| IBIS file stm32mp157xab_lfbga354.ibs
[IBIS ver]   4.2
[File name]   stm32mp157xab_lfbga354.ibs
[File Rev]   2.2
[Date]   07-07-2026
[Source]   Data Created at STMicroelectronics
[Disclaimer]  This information is for modeling purpose only and is
   not guaranted.
   The information is subject to change without notice.
[Copyright]   Copyright 2026 STMicroelectronics Inc.
|   Component stm32mp157xab_lfbga354
[Component] stm32mp157xab_lfbga354
[Manufacturer] STMicroelectronics
[Package]
| variable   typ   min   max
R_pkg  5.94E-01  2.68E-01  8.52E-01
L_pkg  3.75E-09  1.99E-09  5.34E-09
C_pkg  1.24E-12  9.33E-13  5.22E-12
[Pin]   signal_name   model_name
A1  VSS  gnd
A2  PG15  io8_ft_hslv
A3  PD0  io8_ft_hslv
A4  PD1  io8_ft_hslv
A5  PE3  io8_ft_hslv
A6  PG6  io8_ft_hslv
A7  PB3  io8_ft_hslv
A8  PB15  io8_ft_hslv
A9  PC7  io8_ft_hslv
A10  PC9  io8_ft_hslv
A11  PC11  io8_ft_hslv
A12  VDD_Unused  nc
A13  DNU  nc
A14  DNU  nc
A15  DNU  nc
A16  VDD1V2_Unused  nc
A17  DDR_DQ0  PDDRIO_PAD
A18  DDR_DQ1  PDDRIO_PAD
A19  VSS  gnd
B1  PE1  io8_ft
B2  VSS  gnd
B3  PE6  io8_ft_hslv
B4  PD7  io8_ft_hslv
B5  PB7  io8_ft_hslv
B6  VSS  gnd
B7  PE5  io8_ft_hslv
B8  PA8  io8_ft_hslv
B9  PB4  io8_ft_hslv
B10  PD2  io8_ft_hslv
B11  PE4  io8_ft_hslv
B12  VDDA1V8_Unused  nc
B13  DNU  nc
B14  DNU  nc
B15  DNU  nc
B16  VDD1V2_Unused  nc
B17  DDR_DQ3  PDDRIO_PAD
B18  DDR_DQ7  PDDRIO_PAD
B19  DDR_DQS0N  PDIFF_PAD
C1  PE11  io8_ft
C2  PE13  io8_ft_hslv
C3  VSS  gnd
C4  PE0  io8_ft_hslv
C5  PD10  io8_ft_hslv
C6  PD3  io8_ft_hslv
C7  PA15  io8_ft_hslv
C8  PA9  io8_ft_hslv
C9  PB14  io8_ft_hslv
C10  PC12  io8_ft_hslv
C11  PC8  io8_ft_hslv
C12  VSS  nc
C13  VSS  nc
C14  VSS  nc
C15  VSS  nc
C16  VSS  nc
C17  VSS  gnd
C18  DDR_DQM0  PDDRIO_PAD
C19  DDR_DQS0P  PDIFF_PAD
D1  VSS  gnd
D2  PE12  io8_ft_hslv
D3  PE14  io8_ft_hslv
D4  VSS  gnd
D5  VSS  gnd
D6  PD4  io8_ft_hslv
D7  PD5  io8_ft_hslv
D8  VSS  gnd
D9  PB9  io8_ft_hslv
D10  PC6  io8_ft_hslv
D11  PC10  io8_ft_hslv
D12  NJTRST  isudqf
D13  JTDI  isudqf
D14  JTDO-TRACESWO  io8_ft
D15  JTMS-SWDIO  io8_ft
D16  JTCK-SWCLK  isudqf
D17  DDR_DQ5  PDDRIO_PAD
D18  DDR_DQ2  PDDRIO_PAD
D19  DDR_DQ6  PDDRIO_PAD
E1  PE15  io8_ft
E2  VSS  gnd
E3  PD6  io8_ft_hslv
E4  VSS  gnd
E5  VSS  gnd
E6  VSS  gnd
E7  VDDCORE  power
E8  VSS  gnd
E9  VDDCORE  power
E10  VSS  gnd
E11  VDDCORE  power
E12  VSS  gnd
E13  VDDCORE  power
E14  VSS  gnd
E15  VDDQ_DDR  power
E16  VSS  gnd
E17  DDR_A7  PDDRIO_PAD
E18  DDR_DQ4  PDDRIO_PAD
F1  PG12  io8_ft_hslv
F2  PD8  io8_ft
F3  PD14  io8_ft
F4  VDDCORE  power
F5  VSS  gnd
F6  VDDCORE  power
F7  VSS  gnd
F8  VDDCORE  power
F9  VSS  gnd
F10  VDDCORE  power
F11  VSS  gnd
F12  VDDCORE  power
F13  VSS_PLL2  gnd
F14  VDDQ_DDR  power
F15  VSS  gnd
F17  DDR_A13  PDDRIO_PAD
F18  DDR_ZQ  nc
F19  DDR_A3  PDDRIO_PAD
G1  PD15  io8_ft
G2  VSS  gnd
G3  PD9  io8_ft
G4  VSS  gnd
G5  VDDCORE  power
G6  VSS  gnd
G7  VDDCORE  power
G8  VSS  gnd
G9  VDDCORE  power
G10  VSS  gnd
G11  VDDCORE  power
G12  VSS  gnd
G13  VDD_PLL2  power
G14  VSS  gnd
G15  VDDQ_DDR  power
G16  DDR_RESETN  PDDRIO_PAD
G17  DDR_A9  PDDRIO_PAD
G18  DDR_A2  PDDRIO_PAD
G19  DDR_BA0  PDDRIO_PAD
H1  PC14-OSC32_IN  io8_ft
H2  PC15-OSC32_OUT  io8_ft
H3  VBAT  power
H4  VDDCORE  power
H5  VSS  gnd
H6  VDDCORE  power
H7  VSS  gnd
H8  VDDCORE  power
H9  VSS  gnd
H10  VDDCORE  power
H11  VSS  gnd
H12  VDDCORE  power
H13  VSS  gnd
H14  VDDQ_DDR  power
H15  VSS  gnd
H17  DDR_A5  PDDRIO_PAD
H18  DDR_A0  PDDRIO_PAD
H19  DDR_ODT  PDDRIO_PAD
|J1  NRST  ioreset_ft_v33
J1  NRST  nc
J2  NRST_CORE  isudqf
J3  VSS  gnd
J4  VSS_PLL  gnd
J5  VDD_PLL  power
J6  VSS  gnd
J7  VDDCORE  power
J8  VSS  gnd
J9  VDDCORE  power
J10  VSS  gnd
J11  VDDCORE  power
J12  VSS  gnd
J13  VDDCORE  power
J14  VSS  gnd
J15  VDDQ_DDR  power
J16  DDR_BA2  PDDRIO_PAD
J17  DDR_WEN  PDDRIO_PAD
J18  DDR_CSN  PDDRIO_PAD
J19  DDR_DTO1  PDDRIO_PAD
K1  BOOT0  isudqf
K2  VSS  gnd
K3  PC13  io8_ft
K4  BOOT1  isudqf
K5  VSS  gnd
K6  VDD  power
K7  VSS  gnd
K8  VDDCORE  power
K9  VSS  gnd
K10  VDDCORE  power
K11  VSS  gnd
K12  VDDCORE  power
K13  VSS  gnd
K14  VDDQ_DDR  power
K15  VSS  gnd
K17  DDR_CASN  PDDRIO_PAD
K18  DDR_DTO0  PDDRIO_PAD
K19  DDR_CLKN  PDDRIO_PAD
L1  PWR_ON  io8_ft
L2  BOOT2  isudqf
L3  VDD_ANA  nc
L4  VSS_ANA  nc
L5  VDD  power
L6  VSS  gnd
L7  VDD  power
L8  VSS  gnd
L9  VDDCORE  power
L10  VSS  gnd
L11  VDDCORE  power
L12  VSS  gnd
L13  VDDCORE  power
L14  VSS  gnd
L15  VDDQ_DDR  power
L16  DDR_A15  PDDRIO_PAD
L17  DDR_A12  PDDRIO_PAD
L18  DDR_RASN  PDDRIO_PAD
L19  DDR_CLKP  PDDRIO_PAD
M1  PH0-OSC_IN  io8_ft
M2  PH1-OSC_OUT  io8_ft
M3  VREF-  nc
M4  VDDA  nc
M5  VSS  gnd
M6  VDD  power
M7  VSS  gnd
M8  VDD  power
M9  VSS  gnd
M10  VDDCORE  power
M11  VSS  gnd
M12  VDDCORE  power
M13  VSS  gnd
M14  VDDQ_DDR  power
M15  VSS  gnd
M17  DDR_A1  PDDRIO_PAD
M18  DDR_A11  PDDRIO_PAD
M19  DDR_A10  PDDRIO_PAD
N1  PDR_ON_CORE  isudqf
N2  PDR_ON  isudqf
N3  VREF+  nc
N4  VSSA  gnd
N5  VDD  power
N6  VSS  gnd
N7  VDD  power
N8  VSS  gnd
N9  VDD  power
N10  VSS  gnd
N11  VDDCORE  power
N12  VSS  gnd
N13  VDDCORE  power
N14  VSS  gnd
N15  VDDQ_DDR  power
N16  DDR_A6  PDDRIO_PAD
N17  DDR_BA1  PDDRIO_PAD
N18  DDR_A14  PDDRIO_PAD
N19  DDR_ATO  nc
P1  PWR_LP  io8_ft
P2  PA13  io8_ft
P3  PA3  io8_ft
P4  PA5  io8_ft_hslv
P5  VSSA  gnd
P6  VDD  power
P7  VSS  gnd
P8  VDD  power
P9  VSS  gnd
P10  VDD  power
P11  VSS  gnd
P12  VDDCORE  power
P13  VSS  gnd
P14  VDDQ_DDR  power
P15  VSS  gnd
P17  DDR_A4  PDDRIO_PAD
P18  DDR_DQ8  PDDRIO_PAD
P19  DDR_CKE  PDDRIO_PAD
R1  PA14  io8_ft
R2  VSS  gnd
R3  PA0  io8_ft_hslv
R4  PA4  io8_ft
R5  VSSA  gnd
R6  VSS  gnd
R7  VDD_OTP  power
R8  VSS  gnd
R9  VDD  power
R10  VSS  gnd
R11  VDD  power
R12  VSS  gnd
R13  VDDCORE  power
R14  VSS  gnd
R15  VDDQ_DDR  power
R16  VSS  gnd
R17  DDR_A8  PDDRIO_PAD
R18  DDR_DQ10  PDDRIO_PAD
T1  PE2  io8_ft_et_i2c_hslv
T2  PC2  io8_ft_hslv_et
T3  PC3  io8_ft_hslv
T4  VSS  gnd
T5  PA6  io8_ft_hslv
T6  PA7  io8_ft_hslv
T7  PC0  io8_ft_hslv
T8  PB5  io8_ft_hslv_et
T9  PB13  io8_ft_hslv_et
T10  PE7  io8_ft_hslv
T11  PE8  io8_ft_hslv
T12  PB6  io8_ft_i2c_hslv
T13  PB2  io8_ft_hslv
T14  PG9  io8_ft_hslv
T15  BYPASS_REG1V8  isudqf
T16  PA10  io8usb_id_otg20_ft
T17  DDR_DQ9  PDDRIO_PAD
T18  DDR_DQ13  PDDRIO_PAD
T19  DDR_DQS1N  PDIFF_PAD
U1  PG14  io8_ft_hslv_et
U2  PG13  io8_ft_hslv_et
U3  VSS  gnd
U4  PA1  io8_ft_hslv
U5  PF11  io8_ft_hslv
U6  VSS  gnd
U7  PG8  io8_ft_hslv_et
U8  VSS  gnd
U9  PF10  io8_ft_hslv
U10  PF8  io8_ft_hslv
U11  PD12  io8_ft_i2c_hslv
U12  PD13  io8_ft_i2c_hslv
U13  VSS_USBHS  nc
U14  VSS_USBHS  nc
U15  OTG_VBUS  io8usb_vbus_otg20_ft
U16  PA12  io8_i2c_usb_lsfs_bcd_otg20_ft
U17  VSS  gnd
U18  DDR_DM1  PDDRIO_PAD
U19  DDR_DQS1P  PDIFF_PAD
V1  PB11  io8_ft_et_i2c_hslv
V2  PC1  io8_ft_hslv
V3  PB1  io8_ft
V4  PC5  io8_ft
V5  PB12  io8_ft_hslv_et
V6  PG11  io8_ft_hslv_et
V7  PG10  io8_ft_hslv
V8  PD11  io8_ft_hslv
V9  PF6  io8_ft_hslv
V10  PE10  io8_ft_hslv
V11  VDDA1V8_REG  nc
V12  VSS_USBHS  nc
V13  USB_DM2  nc
V14  USB_DP1  nc
V15  VSS_USBHS  nc
V16  USB_RREF  nc
V17  PA11  io8_i2c_usb_lsfs_bcd_otg20_ft
V18  DDR_DQ14  PDDRIO_PAD
V19  DDR_DQ11  PDDRIO_PAD
W1  VSS  gnd
W2  PA2  io8_ft_hslv
W3  PB0  io8_ft
W4  PC4  io8_ft
W5  PB10  io8_ft_i2c_hslv
W6  PB8  io8_ft_et_i2c_hslv
W7  PE9  io8_ft_hslv
W8  PF7  io8_ft_hslv
W9  PF9  io8_ft_hslv
W10  PG7  io8_ft_hslv
W11  VDDA1V1_REG  nc
W12  VDD3V3_USBHS  power
W13  USB_DP2  nc
W14  USB_DM1  nc
W15  VDD3V3_USBFS  power
W16  DDR_VREF  POWER
W17  DDR_DQ15  PDDRIO_PAD
W18  DDR_DQ12  PDDRIO_PAD
W19  VSS  gnd
[Package Model]   500-lfbga-16x16-354-100mhz-181019
[Pin Mapping]   pulldown_ref   pullup_ref   | Comment
A1  VSS  nc
A2  VSS  VDD
A3  VSS  VDD
A4  VSS  VDD
A5  VSS  VDD
A6  VSS  VDD
A7  VSS  VDD
A8  VSS  VDD
A9  VSS  VDD
A10  VSS  VDD
A11  VSS  VDD
A12  nc  nc
A13  nc nc
A14  nc nc
A15  nc nc
A16  nc nc
A17  VSS  VDDQ_DDR
A18  VSS  VDDQ_DDR
A19  VSS  nc
B1  VSS  VDD
B2  VSS  nc
B3  VSS  VDD
B4  VSS  VDD
B5  VSS  VDD
B6  VSS  nc
B7  VSS  VDD
B8  VSS  VDD
B9  VSS  VDD
B10  VSS  VDD
B11  VSS  VDD
B12  nc nc
B13  nc nc
B14  nc nc
B15  nc nc
B16  nc  nc
B17  VSS  VDDQ_DDR
B18  VSS  VDDQ_DDR
B19  VSS  VDDQ_DDR
C1  VSS  VDD
C2  VSS  VDD
C3  VSS  nc
C4  VSS  VDD
C5  VSS  VDD
C6  VSS  VDD
C7  VSS  VDD
C8  VSS  VDD
C9  VSS  VDD
C10  VSS  VDD
C11  VSS  VDD
C12  nc nc
C13  nc nc
C14  nc nc
C15  nc nc
C16  nc nc
C17  VSS  nc
C18  VSS  VDDQ_DDR
C19  VSS  VDDQ_DDR
D1  VSS  nc
D2  VSS  VDD
D3  VSS  VDD
D4  VSS  nc
D5  VSS  nc
D6  VSS  VDD
D7  VSS  VDD
D8  VSS  nc
D9  VSS  VDD
D10  VSS  VDD
D11  VSS  VDD
D12  VSS  VDD
D13  VSS  VDD
D14  VSS  VDD
D15  VSS  VDD
D16  VSS  VDD
D17  VSS  VDDQ_DDR
D18  VSS  VDDQ_DDR
D19  VSS  VDDQ_DDR
E1  VSS  VDD
E2  VSS  nc
E3  VSS  VDD
E4  VSS  nc
E5  VSS  nc
E6  VSS  nc
E7  nc  vddcore
E8  VSS  nc
E9  nc  vddcore
E10  VSS  nc
E11  nc  vddcore
E12  VSS  nc
E13  nc  vddcore
E14  VSS  nc
E15  nc  VDDQ_DDR
E16  VSS  nc
E17  VSS  VDDQ_DDR
E18  VSS  VDDQ_DDR
F1  VSS  VDD
F2  VSS  VDD
F3  VSS  VDD
F4  nc  vddcore
F5  VSS  nc
F6  nc  vddcore
F7  VSS  nc
F8  nc  vddcore
F9  VSS  nc
F10  nc  vddcore
F11  VSS  nc
F12  nc  vddcore
F13  VSS  nc
F14  nc  VDDQ_DDR
F15  VSS  nc
F17  VSS  VDDQ_DDR
F18  nc nc
F19  VSS  VDDQ_DDR
G1  VSS  VDD
G2  VSS  nc
G3  VSS  VDD
G4  VSS  nc
G5  nc  vddcore
G6  VSS  nc
G7  nc  vddcore
G8  VSS  nc
G9  nc  vddcore
G10  VSS  nc
G11  nc  vddcore
G12  VSS  nc
G13  nc  VDD
G14  VSS  nc
G15  nc  VDDQ_DDR
G16  VSS  VDDQ_DDR
G17  VSS  VDDQ_DDR
G18  VSS  VDDQ_DDR
G19  VSS  VDDQ_DDR
H1  nc  nc
H2  nc  nc
H3  nc  VDD_sw
H4  nc  vddcore
H5  VSS  nc
H6  nc  vddcore
H7  VSS  nc
H8  nc  vddcore
H9  VSS  nc
H10  nc  vddcore
H11  VSS  nc
H12  nc  vddcore
H13  VSS  nc
H14  nc  VDDQ_DDR
H15  VSS  nc
H17  VSS  VDDQ_DDR
H18  VSS  VDDQ_DDR
H19  VSS  VDDQ_DDR
J1  nc  nc
J2  VSS  VDD
J3  VSS  nc
J4  VSS  nc
J5  nc  VDD
J6  VSS  nc
J7  nc  vddcore
J8  VSS  nc
J9  nc  vddcore
J10  VSS  nc
J11  nc  vddcore
J12  VSS  nc
J13  nc  vddcore
J14  VSS  nc
J15  nc  VDDQ_DDR
J16  VSS  VDDQ_DDR
J17  VSS  VDDQ_DDR
J18  VSS  VDDQ_DDR
J19  VSS  VDDQ_DDR
K1  VSS  VDD
K2  VSS  nc
K3  nc  nc
K4  VSS  VDD
K5  VSS  nc
K6  nc  VDD
K7  VSS  nc
K8  nc  vddcore
K9  VSS  nc
K10  nc  vddcore
K11  VSS  nc
K12  nc  vddcore
K13  VSS  nc
K14  nc  VDDQ_DDR
K15  VSS  nc
K17  VSS  VDDQ_DDR
K18  VSS  VDDQ_DDR
K19  VSS  VDDQ_DDR
L1  VSS  VDD
L2  VSS  VDD
L3  nc nc
L4  nc nc
L5  nc  VDD
L6  VSS  nc
L7  nc  VDD
L8  VSS  nc
L9  nc  vddcore
L10  VSS  nc
L11  nc  vddcore
L12  VSS  nc
L13  nc  vddcore
L14  VSS  nc
L15  nc  VDDQ_DDR
L16  VSS  VDDQ_DDR
L17  VSS  VDDQ_DDR
L18  VSS  VDDQ_DDR
L19  VSS  VDDQ_DDR
M1  VSS  VDD
M2  VSS  VDD
M3  nc nc
M4  nc nc
M5  VSS  nc
M6  nc  VDD
M7  VSS  nc
M8  nc  VDD
M9  VSS  nc
M10  nc  vddcore
M11  VSS  nc
M12  nc  vddcore
M13  VSS  nc
M14  nc  VDDQ_DDR
M15  VSS  nc
M17  VSS  VDDQ_DDR
M18  VSS  VDDQ_DDR
M19  VSS  VDDQ_DDR
N1  VSS  VDD
N2  VSS  VDD
N3  nc nc
N4  VSS  nc
N5  nc  VDD
N6  VSS  nc
N7  nc  VDD
N8  VSS  nc
N9  nc  VDD
N10  VSS  nc
N11  nc  vddcore
N12  VSS  nc
N13  nc  vddcore
N14  VSS  nc
N15  nc  VDDQ_DDR
N16  VSS  VDDQ_DDR
N17  VSS  VDDQ_DDR
N18  VSS  VDDQ_DDR
N19  nc nc
P1  VSS  VDD
P2  VSS  VDD
P3  VSS  VDD
P4  VSS  VDD
P5  VSS  nc
P6  nc  VDD
P7  VSS  nc
P8  nc  VDD
P9  VSS  nc
P10  nc  VDD
P11  VSS  nc
P12  nc  vddcore
P13  VSS  nc
P14  nc  VDDQ_DDR
P15  VSS  nc
P17  VSS  VDDQ_DDR
P18  VSS  VDDQ_DDR
P19  VSS  VDDQ_DDR
R1  VSS  VDD
R2  VSS  nc
R3  VSS  VDD
R4  VSS  VDD
R5  VSS  nc
R6  VSS  nc
R7  nc  VDD
R8  VSS  nc
R9  nc  VDD
R10  VSS  nc
R11  nc  VDD
R12  VSS  nc
R13  nc  vddcore
R14  VSS  nc
R15  nc  VDDQ_DDR
R16  VSS  nc
R17  VSS  VDDQ_DDR
R18  VSS  VDDQ_DDR
T1  VSS  VDD
T2  VSS  VDD
T3  VSS  VDD
T4  VSS  nc
T5  VSS  VDD
T6  VSS  VDD
T7  VSS  VDD
T8  VSS  VDD
T9  VSS  VDD
T10  VSS  VDD
T11  VSS  VDD
T12  VSS  VDD
T13  VSS  VDD
T14  VSS  VDD
T15  VSS  VDD
T16  VSS  vddusbls  | Depending on IO usage
| T16  VSS  VDD  | Depending on IO usage
T17  VSS  VDDQ_DDR
T18  VSS  VDDQ_DDR
T19  VSS  VDDQ_DDR
U1  VSS  VDD
U2  VSS  VDD
U3  VSS  nc
U4  VSS  VDD
U5  VSS  VDD
U6  VSS  nc
U7  VSS  VDD
U8  VSS  nc
U9  VSS  VDD
U10  VSS  VDD
U11  VSS  VDD
U12  VSS  VDD
U13  nc nc
U14  nc nc
U15  VSS  vddusbls  | Depending on IO usage
| U15  VSS  VDD  | Depending on IO usage
U16  VSS  vddusbls  | Depending on IO usage
| U16  VSS  VDD  | Depending on IO usage
U17  VSS  nc
U18  VSS  VDDQ_DDR
U19  VSS  VDDQ_DDR
V1  VSS  VDD
V2  VSS  VDD
V3  VSS  VDD
V4  VSS  VDD
V5  VSS  VDD
V6  VSS  VDD
V7  VSS  VDD
V8  VSS  VDD
V9  VSS  VDD
V10  VSS  VDD
V11  nc  nc
V12  nc nc
V13  nc nc
V14  nc nc
V15  nc nc
V16  nc nc
V17  VSS  vddusbls  | Depending on IO usage
| V17  VSS  VDD  | Depending on IO usage
V18  VSS  VDDQ_DDR
V19  VSS  VDDQ_DDR
W1  VSS  nc
W2  VSS  VDD
W3  VSS  VDD
W4  VSS  VDD
W5  VSS  VDD
W6  VSS  VDD
W7  VSS  VDD
W8  VSS  VDD
W9  VSS  VDD
W10  VSS  VDD
W11  nc  nc
W12  nc  vddusbhs
W13  nc nc
W14  nc nc
W15  nc  vddusbls
W16  nc  VDDQ_DDR
W17  VSS  VDDQ_DDR
W18  VSS  VDDQ_DDR
W19  VSS  nc
|**********************DIFF PIN*********************************************
[Diff_pin]   inv_pin   vdiff   tdelay_typ   tdelay_min   tdelay_max
   L19   K19   0.320V   0ns   NA   NA   |CK
   C19   B19   0.320V   0ns   NA   NA   |DQS0
   U19   T19   0.320V   0ns   NA   NA   |DQS1
[Model Selector] io8usb_id_otg20_ft
io8_ft_ls_1v2   "GPIO - 5V tolerant - 1.2V range - Low speed"
io8_ft_ms_1v2   "GPIO - 5V tolerant - 1.2V range - Med speed"
io8_ft_hs_1v2   "GPIO - 5V tolerant - 1.2V range - High speed"
io8_ft_fs_1v2   "GPIO - 5V tolerant - 1.2V range - Fast speed"
io8_ft_hs_1v8   "GPIO - 5V tolerant - 1.8V range - High speed"
io8_ft_fs_1v8   "GPIO - 5V tolerant - 1.8V range - Fast speed"
io8_ft_ms_1v8   "GPIO - 5V tolerant - 1.8V range - Med speed"
io8_ft_ls_1v8   "GPIO - 5V tolerant - 1.8V range - Low speed"
io8_ft_hs_3v3   "GPIO - 5V tolerant - 3.3V range - High speed"
io8_ft_fs_3v3   "GPIO - 5V tolerant - 3.3V range - Fast speed"
io8_ft_ms_3v3   "GPIO - 5V tolerant - 3.3V range - Med speed"
io8_ft_ls_3v3   "GPIO - 5V tolerant - 3.3V range - Low speed"
[Model Selector] io8usb_vbus_otg20_ft
io8_ft_ls_1v2   "GPIO - 5V tolerant - 1.2V range - Low speed"
io8_ft_ms_1v2   "GPIO - 5V tolerant - 1.2V range - Med speed"
io8_ft_hs_1v2   "GPIO - 5V tolerant - 1.2V range - High speed"
io8_ft_fs_1v2   "GPIO - 5V tolerant - 1.2V range - Fast speed"
io8_ft_hs_1v8   "GPIO - 5V tolerant - 1.8V range - High speed"
io8_ft_fs_1v8   "GPIO - 5V tolerant - 1.8V range - Fast speed"
io8_ft_ms_1v8   "GPIO - 5V tolerant - 1.8V range - Med speed"
io8_ft_ls_1v8   "GPIO - 5V tolerant - 1.8V range - Low speed"
io8_ft_hs_3v3   "GPIO - 5V tolerant - 3.3V range - High speed"
io8_ft_fs_3v3   "GPIO - 5V tolerant - 3.3V range - Fast speed"
io8_ft_ms_3v3   "GPIO - 5V tolerant - 3.3V range - Med speed"
io8_ft_ls_3v3   "GPIO - 5V tolerant - 3.3V range - Low speed"
[Model Selector] io8_ft
io8_ft_ls_1v2   "GPIO - 5V tolerant - 1.2V range - Low speed"
io8_ft_ms_1v2   "GPIO - 5V tolerant - 1.2V range - Med speed"
io8_ft_hs_1v2   "GPIO - 5V tolerant - 1.2V range - High speed"
io8_ft_fs_1v2   "GPIO - 5V tolerant - 1.2V range - Fast speed"
io8_ft_hs_1v8   "GPIO - 5V tolerant - 1.8V range - High speed"
io8_ft_fs_1v8   "GPIO - 5V tolerant - 1.8V range - Fast speed"
io8_ft_ms_1v8   "GPIO - 5V tolerant - 1.8V range - Med speed"
io8_ft_ls_1v8   "GPIO - 5V tolerant - 1.8V range - Low speed"
io8_ft_hs_3v3   "GPIO - 5V tolerant - 3.3V range - High speed"
io8_ft_fs_3v3   "GPIO - 5V tolerant - 3.3V range - Fast speed"
io8_ft_ms_3v3   "GPIO - 5V tolerant - 3.3V range - Med speed"
io8_ft_ls_3v3   "GPIO - 5V tolerant - 3.3V range - Low speed"
[Model Selector] io8_ft_hslv
io8_ft_ls_1v2   "GPIO - 5V tolerant - 1.2V range - Low speed"
io8_ft_ms_1v2   "GPIO - 5V tolerant - 1.2V range - Med speed"
io8_ft_hs_1v2   "GPIO - 5V tolerant - 1.2V range - High speed"
io8_ft_fs_1v2   "GPIO - 5V tolerant - 1.2V range - Fast speed"
io8_ft_hs_1v8   "GPIO - 5V tolerant - 1.8V range - High speed"
io8_ft_fs_1v8   "GPIO - 5V tolerant - 1.8V range - Fast speed"
io8_ft_ms_1v8   "GPIO - 5V tolerant - 1.8V range - Med speed"
io8_ft_ls_1v8   "GPIO - 5V tolerant - 1.8V range - Low speed"
io8_ft_hs_3v3   "GPIO - 5V tolerant - 3.3V range - High speed"
io8_ft_fs_3v3   "GPIO - 5V tolerant - 3.3V range - Fast speed"
io8_ft_ms_3v3   "GPIO - 5V tolerant - 3.3V range - Med speed"
io8_ft_ls_3v3   "GPIO - 5V tolerant - 3.3V range - Low speed"
io8_ft_hslv_hs_1v2   "GPIO - hslv opt - 5V tolerant - 1.2V range - High speed"
io8_ft_hslv_fs_1v2   "GPIO - hslv opt - 5V tolerant - 1.2V range - Fast speed"
io8_ft_hslv_ms_1v2   "GPIO - hslv opt - 5V tolerant - 1.2V range - Med speed"
io8_ft_hslv_ls_1v2   "GPIO - hslv opt - 5V tolerant - 1.2V range - Low speed"
io8_ft_hslv_hs_1v8   "GPIO - hslv opt - 5V tolerant - 1.8V range - High speed"
io8_ft_hslv_fs_1v8   "GPIO - hslv opt - 5V tolerant - 1.8V range - Fast speed"
io8_ft_hslv_ms_1v8   "GPIO - hslv opt - 5V tolerant - 1.8V range - Med speed"
io8_ft_hslv_ls_1v8   "GPIO - hslv opt - 5V tolerant - 1.8V range - Low speed"
io8_ft_hslv_hs_2v5   "GPIO - hslv opt - 5V tolerant - 2.5V range - High speed"
io8_ft_hslv_fs_2v5   "GPIO - hslv opt - 5V tolerant - 2.5V range - Fast speed"
io8_ft_hslv_ms_2v5   "GPIO - hslv opt - 5V tolerant - 2.5V range - Med speed"
io8_ft_hslv_ls_2v5   "GPIO - hslv opt - 5V tolerant - 2.5V range - Low speed"
[Model Selector] io8_ft_hslv_et
io8_ft_et_ls_1v2   "GPIO - Ethernet - 5V tol - 1.2V range - Low speed"
io8_ft_et_ms_1v2   "GPIO - Ethernet - 5V tol - 1.2V range - Med speed"
io8_ft_et_hs_1v2   "GPIO - Ethernet - 5V tol - 1.2V range - High speed"
io8_ft_et_fs_1v2   "GPIO - Ethernet - 5V tol - 1.2V range - Fast speed"
io8_ft_et_hs_1v8   "GPIO - Ethernet - 5V tol - 1.8V range - High speed"
io8_ft_et_fs_1v8   "GPIO - Ethernet - 5V tol - 1.8V range - Fast speed"
io8_ft_et_ms_1v8   "GPIO - Ethernet - 5V tol - 1.8V range - Med speed"
io8_ft_et_ls_1v8   "GPIO - Ethernet - 5V tol - 1.8V range - Low speed"
io8_ft_et_hs_3v3   "GPIO - Ethernet - 5V tol - 3.3V range - High speed"
io8_ft_et_fs_3v3   "GPIO - Ethernet - 5V tol - 3.3V range - Fast speed"
io8_ft_et_ms_3v3   "GPIO - Ethernet - 5V tol - 3.3V range - Med speed"
io8_ft_et_ls_3v3   "GPIO - Ethernet - 5V tol - 3.3V range - Low speed"
io8_ft_et_hslv_ls_1v2   "GPIO - hslv opt - Ethernet - 5V tol - 1.2V range - Low speed"
io8_ft_et_hslv_hs_1v2   "GPIO - hslv opt - Ethernet - 5V tol - 1.2V range - High speed"
io8_ft_et_hslv_fs_1v2   "GPIO - hslv opt - Ethernet - 5V tol - 1.2V range - Fast speed"
io8_ft_et_hslv_ms_1v2   "GPIO - hslv opt - Ethernet - 5V tol - 1.2V range - Med speed"
io8_ft_et_hslv_ls_1v8   "GPIO - hslv opt - Ethernet - 5V tol - 1.8V range - Low speed"
io8_ft_et_hslv_hs_1v8   "GPIO - hslv opt - Ethernet - 5V tol - 1.8V range - High speed"
io8_ft_et_hslv_fs_1v8   "GPIO - hslv opt - Ethernet - 5V tol - 1.2V range - Fast speed"
io8_ft_et_hslv_ms_1v8   "GPIO - hslv opt - Ethernet - 5V tol - 1.8V range - Med speed"
io8_ft_et_hslv_hs_2v5   "GPIO - hslv opt - Ethernet - 5V tol - 2.5V range - High speed"
io8_ft_et_hslv_fs_2v5   "GPIO - hslv opt - Ethernet - 5V tol - 2.5V range - Fast speed"
io8_ft_et_hslv_ms_2v5   "GPIO - hslv opt - Ethernet - 5V tol - 2.5V range - Med speed"
io8_ft_et_hslv_ls_2v5   "GPIO - hslv opt - Ethernet - 5V tol - 2.5V range - Low speed"
[Model Selector] io8_ft_et_i2c_hslv
io8_ft_et_ls_1v2   "GPIO - 5V tol - 1.2V range - Low speed"
io8_ft_et_ms_1v2   "GPIO - 5V tol - 1.2V range - Med speed"
io8_ft_et_hs_1v2   "GPIO - 5V tol - 1.2V range - High speed"
io8_ft_et_fs_1v2   "GPIO - 5V tol - 1.2V range - Fast speed"
io8_ft_et_hs_1v8   "GPIO - 5V tol - 1.8V range - High speed"
io8_ft_et_fs_1v8   "GPIO - 5V tol - 1.8V range - Fast speed"
io8_ft_et_ms_1v8   "GPIO - 5V tol - 1.8V range - Med speed"
io8_ft_et_ls_1v8   "GPIO - 5V tol - 1.8V range - Low speed"
io8_ft_et_hs_3v3   "GPIO - 5V tol - 3.3V range - High speed"
io8_ft_et_fs_3v3   "GPIO - 5V tol - 3.3V range - Fast speed"
io8_ft_et_ms_3v3   "GPIO - 5V tol - 3.3V range - Med speed"
io8_ft_et_ls_3v3   "GPIO - 5V tol - 3.3V range - Low speed"
io8_ft_et_hslv_ls_1v2   "GPIO - hslv opt -Ethernet - 5V tol - 1.2V range - Low speed"
io8_ft_et_hslv_hs_1v2   "GPIO - hslv opt -Ethernet - 5V tol - 1.2V range - High speed"
io8_ft_et_hslv_fs_1v2   "GPIO - hslv opt -Ethernet - 5V tol - 1.2V range - Fast speed"
io8_ft_et_hslv_ms_1v2   "GPIO - hslv opt -Ethernet - 5V tol - 1.2V range - Med speed"
io8_ft_et_hslv_ls_1v8   "GPIO - hslv opt -Ethernet - 5V tol - 1.8V range - Low speed"
io8_ft_et_hslv_hs_1v8   "GPIO - hslv opt -Ethernet - 5V tol - 1.8V range - High speed"
io8_ft_et_hslv_fs_1v8   "GPIO - hslv opt -Ethernet - 5V tol - 1.2V range - Fast speed"
io8_ft_et_hslv_ms_1v8   "GPIO - hslv opt -Ethernet - 5V tol - 1.8V range - Med speed"
io8_ft_et_hslv_hs_2v5   "GPIO - hslv opt -Ethernet - 5V tol - 2.5V range - High speed"
io8_ft_et_hslv_fs_2v5   "GPIO - hslv opt  -Ethernet- 5V tol - 2.5V range - Fast speed"
io8_ft_et_hslv_ms_2v5   "GPIO - hslv opt -Ethernet - 5V tol - 2.5V range - Med speed"
io8_ft_et_hslv_ls_2v5   "GPIO - hslv opt -Ethernet - 5V tol - 2.5V range - Low speed"
io8_ft_i2c_1v2   "GPIO - 5V tolerant - 1.2V range - Open drain"
io8_ft_i2c_1v8   "GPIO - 5V tolerant - 1.8V range - Open drain"
io8_ft_i2c_3v3   "GPIO - 5V tolerant - 3.3V range - Open drain"
io8_ft_i2c_hslv_1v2   "GPIO - hslv opt - 5V tolerant - 1.2V range - Open drain"
io8_ft_i2c_hslv_1v8   "GPIO - hslv opt - 5V tolerant - 1.8V range - Open drain"
io8_ft_i2c_hslv_2v5   "GPIO - hslv opt - 5V tolerant - 2.5V range - Open drain"
[Model Selector] io8_ft_i2c_hslv
io8_ft_ls_1v2   "GPIO - 5V tolerant - 1.2V range - Low speed"
io8_ft_ms_1v2   "GPIO - 5V tolerant - 1.2V range - Med speed"
io8_ft_hs_1v2   "GPIO - 5V tolerant - 1.2V range - High speed"
io8_ft_fs_1v2   "GPIO - 5V tolerant - 1.2V range - Fast speed"
io8_ft_hs_1v8   "GPIO - 5V tolerant - 1.8V range - High speed"
io8_ft_fs_1v8   "GPIO - 5V tolerant - 1.8V range - Fast speed"
io8_ft_ms_1v8   "GPIO - 5V tolerant - 1.8V range - Med speed"
io8_ft_ls_1v8   "GPIO - 5V tolerant - 1.8V range - Low speed"
io8_ft_hs_3v3   "GPIO - 5V tolerant - 3.3V range - High speed"
io8_ft_fs_3v3   "GPIO - 5V tolerant - 3.3V range - Fast speed"
io8_ft_ms_3v3   "GPIO - 5V tolerant - 3.3V range - Med speed"
io8_ft_ls_3v3   "GPIO - 5V tolerant - 3.3V range - Low speed"
io8_ft_hslv_hs_1v2   "GPIO - hslv opt - 5V tolerant - 1.2V range - High speed"
io8_ft_hslv_fs_1v2   "GPIO - hslv opt - 5V tolerant - 1.2V range - Fast speed"
io8_ft_hslv_ms_1v2   "GPIO - hslv opt - 5V tolerant - 1.2V range - Med speed"
io8_ft_hslv_ls_1v2   "GPIO - hslv opt - 5V tolerant - 1.2V range - Low speed"
io8_ft_hslv_hs_1v8   "GPIO - hslv opt - 5V tolerant - 1.8V range - High speed"
io8_ft_hslv_fs_1v8   "GPIO - hslv opt - 5V tolerant - 1.8V range - Fast speed"
io8_ft_hslv_ms_1v8   "GPIO - hslv opt - 5V tolerant - 1.8V range - Med speed"
io8_ft_hslv_ls_1v8   "GPIO - hslv opt - 5V tolerant - 1.8V range - Low speed"
io8_ft_hslv_hs_2v5   "GPIO - hslv opt - 5V tolerant - 2.5V range - High speed"
io8_ft_hslv_fs_2v5   "GPIO - hslv opt - 5V tolerant - 2.5V range - Fast speed"
io8_ft_hslv_ms_2v5   "GPIO - hslv opt - 5V tolerant - 2.5V range - Med speed"
io8_ft_hslv_ls_2v5   "GPIO - hslv opt - 5V tolerant - 2.5V range - Low speed"
io8_ft_i2c_1v2   "GPIO - 5V tolerant - 1.2V range - Open drain"
io8_ft_i2c_1v8   "GPIO - 5V tolerant - 1.8V range - Open drain"
io8_ft_i2c_3v3   "GPIO - 5V tolerant - 3.3V range - Open drain"
io8_ft_i2c_hslv_1v2   "GPIO - hslv opt - 5V tolerant - 1.2V range - Open drain"
io8_ft_i2c_hslv_1v8   "GPIO - hslv opt - 5V tolerant - 1.8V range - Open drain"
io8_ft_i2c_hslv_2v5   "GPIO - hslv opt - 5V tolerant - 2.5V range - Open drain"
[Model Selector] io8_i2c_usb_lsfs_bcd_otg20_ft
io8_ft_ls_1v2   "GPIO - 5V tolerant - 1.2V range - Low speed"
io8_ft_ms_1v2   "GPIO - 5V tolerant - 1.2V range - Med speed"
io8_ft_hs_1v2   "GPIO - 5V tolerant - 1.2V range - High speed"
io8_ft_fs_1v2   "GPIO - 5V tolerant - 1.2V range - Fast speed"
io8_ft_hs_1v8   "GPIO - 5V tolerant - 1.8V range - High speed"
io8_ft_fs_1v8   "GPIO - 5V tolerant - 1.8V range - Fast speed"
io8_ft_ms_1v8   "GPIO - 5V tolerant - 1.8V range - Med speed"
io8_ft_ls_1v8   "GPIO - 5V tolerant - 1.8V range - Low speed"
io8_ft_hs_3v3   "GPIO - 5V tolerant - 3.3V range - High speed"
io8_ft_fs_3v3   "GPIO - 5V tolerant - 3.3V range - Fast speed"
io8_ft_ms_3v3   "GPIO - 5V tolerant - 3.3V range - Med speed"
io8_ft_ls_3v3   "GPIO - 5V tolerant - 3.3V range - Low speed"
io8_ft_i2c_1v2   "GPIO - 5V tolerant - 1.2V range - Open drain"
io8_ft_i2c_1v8   "GPIO - 5V tolerant - 1.8V range - Open drain"
io8_ft_i2c_3v3   "GPIO - 5V tolerant - 3.3V range - Open drain"
io8usb_ft_hs_3v3   "USB full speed"
io8usb_ft_ls_3v3   "USB low speed"
|[Model Selector] ioreset_ft_v33
|ioreset_ft_v33_1v2   "Reset PAD. 5V tolerant. 1.2V range"
|ioreset_ft_v33_1v8   "Reset PAD. 5V tolerant. 1.8V range"
|ioreset_ft_v33_3v3   "Reset PAD. 5V tolerant. 3.3V range"
[Model Selector] isudqf
isudqf_1v2   "Input Buffer - 5V tolerant - 1.2V range"
isudqf_1v8   "Input Buffer - 5V tolerant - 1.8V range"
isudqf_3v3   "Input Buffer - 5V tolerant - 3.3V range"
[Model Selector] PDIFF_PAD
MSD_D3RF2_18   DDR2 MSD_D3R_PDIFF Z0=18-Ohm
MSD_D3RF2_40   DDR2 MSD_D3R_PDIFF Z0=40-Ohm
MSD_D3RF2_48   DDR2 MSD_D3R_PDIFF Z0=48-Ohm
MSD_D3RF2_ODT150   DDR2 MSD_D3R_PDIFF cell 150-Ohm ODT Receiver
MSD_D3RF2_ODT50   DDR2 MSD_D3R_PDIFF cell 50-Ohm ODT Receiver
MSD_D3RF2_ODT75   DDR2 MSD_D3R_PDIFF cell 75-Ohm ODT Receiver
MSD_D3RF2_ODTOFF   DDR2 MSD_D3R_PDIFF cell ODT off Receiver
MSD_D3RF3_34   DDR3 MSD_D3R_PDIFF cell  Z0=34-Ohm
MSD_D3RF3_40   DDR3 MSD_D3R_PDIFF cell  Z0=40-Ohm
MSD_D3RF3_48   DDR3 MSD_D3R_PDIFF cell  Z0=48-Ohm
MSD_D3RF3L_34   DDR3L MSD_D3R_PDIFF cell  Z0=34-Ohm
MSD_D3RF3L_40   DDR3L MSD_D3R_PDIFF cell  Z0=40-Ohm
MSD_D3RF3L_48   DDR3L MSD_D3R_PDIFF cell  Z0=48-Ohm
MSD_D3RF3L_ODT120   DDR3L MSD_D3R_PDIFF cell 120-Ohm ODT Receiver
MSD_D3RF3L_ODT40   DDR3L MSD_D3R_PDIFF cell 40-Ohm ODT Receiver
MSD_D3RF3L_ODT60   DDR3L MSD_D3R_PDIFF cell 60-Ohm ODT Receiver
MSD_D3RF3L_ODTOFF   DDR3L MSD_D3R_PDIFF cell ODT off Receiver
MSD_D3RF3_ODT120   DDR3 MSD_D3R_PDIFF cell 120-Ohm ODT Receiver
MSD_D3RF3_ODT40   DDR3 MSD_D3R_PDIFF cell 40-Ohm ODT Receiver
MSD_D3RF3_ODT60   DDR3 MSD_D3R_PDIFF cell 60-Ohm ODT Receiver
MSD_D3RF3_ODTOFF   DDR3 MSD_D3R_PDIFF cell ODT off Receiver
MSD_D3RFL2_34   LPDDR2 MSD_D3R_PDIFF cell  Z0=34-Ohm
MSD_D3RFL2_40   LPDDR2 MSD_D3R_PDIFF cell  Z0=40-Ohm
MSD_D3RFL2_48   LPDDR2 MSD_D3R_PDIFF cell  Z0=48-Ohm
MSD_D3RFL2_60   LPDDR2 MSD_D3R_PDIFF cell  Z0=60-Ohm
MSD_D3RFL2_80   LPDDR2 MSD_D3R_PDIFF cell  Z0=80-Ohm
MSD_D3RFL2_ODTOFF   LPDDR2 MSD_D3R_PDIFF cell ODT off Receiver
MSD_D3RFL_48   LPDDR MSD_D3R_PDIFF cell  Z0=48-Ohm
MSD_D3RFL_ODTOFF   LPDDR MSD_D3R_PDIFF cell ODT off Receiver
MSD_D3RF2_18_OPEN   DDR2 MSD_D3R_PDIFF_PDQSR Z0=18-Ohm
MSD_D3RF2_40_OPEN   DDR2 MSD_D3R_PDIFF_PDQSR Z0=40-Ohm
MSD_D3RF2_48_OPEN   DDR2 MSD_D3R_PDIFF_PDQSR Z0=48-Ohm
MSD_D3RF2_18_PD344   DDR2 MSD_D3R_PDIFF_PDQSR Z0=18-Ohm
MSD_D3RF2_40_PD344   DDR2 MSD_D3R_PDIFF_PDQSR Z0=40-Ohm
MSD_D3RF2_48_PD344   DDR2 MSD_D3R_PDIFF_PDQSR Z0=48-Ohm
MSD_D3RF2_18_PD393   DDR2 MSD_D3R_PDIFF_PDQSR Z0=18-Ohm
MSD_D3RF2_40_PD393   DDR2 MSD_D3R_PDIFF_PDQSR Z0=40-Ohm
MSD_D3RF2_48_PD393   DDR2 MSD_D3R_PDIFF_PDQSR Z0=48-Ohm
MSD_D3RF2_18_PD458   DDR2 MSD_D3R_PDIFF_PDQSR Z0=18-Ohm
MSD_D3RF2_40_PD458   DDR2 MSD_D3R_PDIFF_PDQSR Z0=40-Ohm
MSD_D3RF2_48_PD458   DDR2 MSD_D3R_PDIFF_PDQSR Z0=48-Ohm
MSD_D3RF2_18_PD500   DDR2 MSD_D3R_PDIFF_PDQSR Z0=18-Ohm
MSD_D3RF2_40_PD500   DDR2 MSD_D3R_PDIFF_PDQSR Z0=40-Ohm
MSD_D3RF2_48_PD500   DDR2 MSD_D3R_PDIFF_PDQSR Z0=48-Ohm
MSD_D3RF2_18_PD550   DDR2 MSD_D3R_PDIFF_PDQSR Z0=18-Ohm
MSD_D3RF2_40_PD550   DDR2 MSD_D3R_PDIFF_PDQSR Z0=40-Ohm
MSD_D3RF2_48_PD550   DDR2 MSD_D3R_PDIFF_PDQSR Z0=48-Ohm
MSD_D3RF2_18_PD611   DDR2 MSD_D3R_PDIFF_PDQSR Z0=18-Ohm
MSD_D3RF2_40_PD611   DDR2 MSD_D3R_PDIFF_PDQSR Z0=40-Ohm
MSD_D3RF2_48_PD611   DDR2 MSD_D3R_PDIFF_PDQSR Z0=48-Ohm
MSD_D3RF2_18_PD688   DDR2 MSD_D3R_PDIFF_PDQSR Z0=18-Ohm
MSD_D3RF2_40_PD688   DDR2 MSD_D3R_PDIFF_PDQSR Z0=40-Ohm
MSD_D3RF2_48_PD688   DDR2 MSD_D3R_PDIFF_PDQSR Z0=48-Ohm
MSD_D3RF2_18_PU344   DDR2 MSD_D3R_PDIFF_PDQSR Z0=18-Ohm
MSD_D3RF2_40_PU344   DDR2 MSD_D3R_PDIFF_PDQSR Z0=40-Ohm
MSD_D3RF2_48_PU344   DDR2 MSD_D3R_PDIFF_PDQSR Z0=48-Ohm
MSD_D3RF2_18_PU393   DDR2 MSD_D3R_PDIFF_PDQSR Z0=18-Ohm
MSD_D3RF2_40_PU393   DDR2 MSD_D3R_PDIFF_PDQSR Z0=40-Ohm
MSD_D3RF2_48_PU393   DDR2 MSD_D3R_PDIFF_PDQSR Z0=48-Ohm
MSD_D3RF2_18_PU458   DDR2 MSD_D3R_PDIFF_PDQSR Z0=18-Ohm
MSD_D3RF2_40_PU458   DDR2 MSD_D3R_PDIFF_PDQSR Z0=40-Ohm
MSD_D3RF2_48_PU458   DDR2 MSD_D3R_PDIFF_PDQSR Z0=48-Ohm
MSD_D3RF2_18_PU500   DDR2 MSD_D3R_PDIFF_PDQSR Z0=18-Ohm
MSD_D3RF2_40_PU500   DDR2 MSD_D3R_PDIFF_PDQSR Z0=40-Ohm
MSD_D3RF2_48_PU500   DDR2 MSD_D3R_PDIFF_PDQSR Z0=48-Ohm
MSD_D3RF2_18_PU550   DDR2 MSD_D3R_PDIFF_PDQSR Z0=18-Ohm
MSD_D3RF2_40_PU550   DDR2 MSD_D3R_PDIFF_PDQSR Z0=40-Ohm
MSD_D3RF2_48_PU550   DDR2 MSD_D3R_PDIFF_PDQSR Z0=48-Ohm
MSD_D3RF2_18_PU611   DDR2 MSD_D3R_PDIFF_PDQSR Z0=18-Ohm
MSD_D3RF2_40_PU611   DDR2 MSD_D3R_PDIFF_PDQSR Z0=40-Ohm
MSD_D3RF2_48_PU611   DDR2 MSD_D3R_PDIFF_PDQSR Z0=48-Ohm
MSD_D3RF2_18_PU688   DDR2 MSD_D3R_PDIFF_PDQSR Z0=18-Ohm
MSD_D3RF2_40_PU688   DDR2 MSD_D3R_PDIFF_PDQSR Z0=40-Ohm
MSD_D3RF2_48_PU688   DDR2 MSD_D3R_PDIFF_PDQSR Z0=48-Ohm
MSD_D3RF2_18_PWRDWN   DDR2 MSD_D3R_PDIFF_PDQSR Z0=18-Ohm
MSD_D3RF2_40_PWRDWN   DDR2 MSD_D3R_PDIFF_PDQSR Z0=40-Ohm
MSD_D3RF2_48_PWRDWN   DDR2 MSD_D3R_PDIFF_PDQSR Z0=48-Ohm
MSD_D3RF3_34_OPEN   DDR3 MSD_D3R_PDIFF_PDQSR cell  Z0=34-Ohm
MSD_D3RF3_40_OPEN   DDR3 MSD_D3R_PDIFF_PDQSR cell  Z0=40-Ohm
MSD_D3RF3_48_OPEN   DDR3 MSD_D3R_PDIFF_PDQSR cell  Z0=48-Ohm
MSD_D3RF3_34_PD344   DDR3 MSD_D3R_PDIFF_PDQSR cell  Z0=34-Ohm
MSD_D3RF3_40_PD344   DDR3 MSD_D3R_PDIFF_PDQSR cell  Z0=40-Ohm
MSD_D3RF3_48_PD344   DDR3 MSD_D3R_PDIFF_PDQSR cell  Z0=48-Ohm
MSD_D3RF3_34_PD393   DDR3 MSD_D3R_PDIFF_PDQSR cell  Z0=34-Ohm
MSD_D3RF3_40_PD393   DDR3 MSD_D3R_PDIFF_PDQSR cell  Z0=40-Ohm
MSD_D3RF3_48_PD393   DDR3 MSD_D3R_PDIFF_PDQSR cell  Z0=48-Ohm
MSD_D3RF3_34_PD458   DDR3 MSD_D3R_PDIFF_PDQSR cell  Z0=34-Ohm
MSD_D3RF3_40_PD458   DDR3 MSD_D3R_PDIFF_PDQSR cell  Z0=40-Ohm
MSD_D3RF3_48_PD458   DDR3 MSD_D3R_PDIFF_PDQSR cell  Z0=48-Ohm
MSD_D3RF3_34_PD500   DDR3 MSD_D3R_PDIFF_PDQSR cell  Z0=34-Ohm
MSD_D3RF3_40_PD500   DDR3 MSD_D3R_PDIFF_PDQSR cell  Z0=40-Ohm
MSD_D3RF3_48_PD500   DDR3 MSD_D3R_PDIFF_PDQSR cell  Z0=48-Ohm
MSD_D3RF3_34_PD550   DDR3 MSD_D3R_PDIFF_PDQSR cell  Z0=34-Ohm
MSD_D3RF3_40_PD550   DDR3 MSD_D3R_PDIFF_PDQSR cell  Z0=40-Ohm
MSD_D3RF3_48_PD550   DDR3 MSD_D3R_PDIFF_PDQSR cell  Z0=48-Ohm
MSD_D3RF3_34_PD611   DDR3 MSD_D3R_PDIFF_PDQSR cell  Z0=34-Ohm
MSD_D3RF3_40_PD611   DDR3 MSD_D3R_PDIFF_PDQSR cell  Z0=40-Ohm
MSD_D3RF3_48_PD611   DDR3 MSD_D3R_PDIFF_PDQSR cell  Z0=48-Ohm
MSD_D3RF3_34_PD688   DDR3 MSD_D3R_PDIFF_PDQSR cell  Z0=34-Ohm
MSD_D3RF3_40_PD688   DDR3 MSD_D3R_PDIFF_PDQSR cell  Z0=40-Ohm
MSD_D3RF3_48_PD688   DDR3 MSD_D3R_PDIFF_PDQSR cell  Z0=48-Ohm
MSD_D3RF3_34_PU344   DDR3 MSD_D3R_PDIFF_PDQSR cell  Z0=34-Ohm
MSD_D3RF3_40_PU344   DDR3 MSD_D3R_PDIFF_PDQSR cell  Z0=40-Ohm
MSD_D3RF3_48_PU344   DDR3 MSD_D3R_PDIFF_PDQSR cell  Z0=48-Ohm
MSD_D3RF3_34_PU393   DDR3 MSD_D3R_PDIFF_PDQSR cell  Z0=34-Ohm
MSD_D3RF3_40_PU393   DDR3 MSD_D3R_PDIFF_PDQSR cell  Z0=40-Ohm
MSD_D3RF3_48_PU393   DDR3 MSD_D3R_PDIFF_PDQSR cell  Z0=48-Ohm
MSD_D3RF3_34_PU458   DDR3 MSD_D3R_PDIFF_PDQSR cell  Z0=34-Ohm
MSD_D3RF3_40_PU458   DDR3 MSD_D3R_PDIFF_PDQSR cell  Z0=40-Ohm
MSD_D3RF3_48_PU458   DDR3 MSD_D3R_PDIFF_PDQSR cell  Z0=48-Ohm
MSD_D3RF3_34_PU500   DDR3 MSD_D3R_PDIFF_PDQSR cell  Z0=34-Ohm
MSD_D3RF3_40_PU500   DDR3 MSD_D3R_PDIFF_PDQSR cell  Z0=40-Ohm
MSD_D3RF3_48_PU500   DDR3 MSD_D3R_PDIFF_PDQSR cell  Z0=48-Ohm
MSD_D3RF3_34_PU550   DDR3 MSD_D3R_PDIFF_PDQSR cell  Z0=34-Ohm
MSD_D3RF3_40_PU550   DDR3 MSD_D3R_PDIFF_PDQSR cell  Z0=40-Ohm
MSD_D3RF3_48_PU550   DDR3 MSD_D3R_PDIFF_PDQSR cell  Z0=48-Ohm
MSD_D3RF3_34_PU611   DDR3 MSD_D3R_PDIFF_PDQSR cell  Z0=34-Ohm
MSD_D3RF3_40_PU611   DDR3 MSD_D3R_PDIFF_PDQSR cell  Z0=40-Ohm
MSD_D3RF3_48_PU611   DDR3 MSD_D3R_PDIFF_PDQSR cell  Z0=48-Ohm
MSD_D3RF3_34_PU688   DDR3 MSD_D3R_PDIFF_PDQSR cell  Z0=34-Ohm
MSD_D3RF3_40_PU688   DDR3 MSD_D3R_PDIFF_PDQSR cell  Z0=40-Ohm
MSD_D3RF3_48_PU688   DDR3 MSD_D3R_PDIFF_PDQSR cell  Z0=48-Ohm
MSD_D3RF3_34_PWRDWN   DDR3 MSD_D3R_PDIFF_PDQSR cell  Z0=34-Ohm
MSD_D3RF3_40_PWRDWN   DDR3 MSD_D3R_PDIFF_PDQSR cell  Z0=40-Ohm
MSD_D3RF3_48_PWRDWN   DDR3 MSD_D3R_PDIFF_PDQSR cell  Z0=48-Ohm
MSD_D3RF3L_34_OPEN   DDR3L MSD_D3R_PDIFF_PDQSR cell  Z0=34-Ohm
MSD_D3RF3L_40_OPEN   DDR3L MSD_D3R_PDIFF_PDQSR cell  Z0=40-Ohm
MSD_D3RF3L_48_OPEN   DDR3L MSD_D3R_PDIFF_PDQSR cell  Z0=48-Ohm
MSD_D3RF3L_34_PD344   DDR3L MSD_D3R_PDIFF_PDQSR cell  Z0=34-Ohm
MSD_D3RF3L_40_PD344   DDR3L MSD_D3R_PDIFF_PDQSR cell  Z0=40-Ohm
MSD_D3RF3L_48_PD344   DDR3L MSD_D3R_PDIFF_PDQSR cell  Z0=48-Ohm
MSD_D3RF3L_34_PD393   DDR3L MSD_D3R_PDIFF_PDQSR cell  Z0=34-Ohm
MSD_D3RF3L_40_PD393   DDR3L MSD_D3R_PDIFF_PDQSR cell  Z0=40-Ohm
MSD_D3RF3L_48_PD393   DDR3L MSD_D3R_PDIFF_PDQSR cell  Z0=48-Ohm
MSD_D3RF3L_34_PD458   DDR3L MSD_D3R_PDIFF_PDQSR cell  Z0=34-Ohm
MSD_D3RF3L_40_PD458   DDR3L MSD_D3R_PDIFF_PDQSR cell  Z0=40-Ohm
MSD_D3RF3L_48_PD458   DDR3L MSD_D3R_PDIFF_PDQSR cell  Z0=48-Ohm
MSD_D3RF3L_34_PD500   DDR3L MSD_D3R_PDIFF_PDQSR cell  Z0=34-Ohm
MSD_D3RF3L_40_PD500   DDR3L MSD_D3R_PDIFF_PDQSR cell  Z0=40-Ohm
MSD_D3RF3L_48_PD500   DDR3L MSD_D3R_PDIFF_PDQSR cell  Z0=48-Ohm
MSD_D3RF3L_34_PD550   DDR3L MSD_D3R_PDIFF_PDQSR cell  Z0=34-Ohm
MSD_D3RF3L_40_PD550   DDR3L MSD_D3R_PDIFF_PDQSR cell  Z0=40-Ohm
MSD_D3RF3L_48_PD550   DDR3L MSD_D3R_PDIFF_PDQSR cell  Z0=48-Ohm
MSD_D3RF3L_34_PD611   DDR3L MSD_D3R_PDIFF_PDQSR cell  Z0=34-Ohm
MSD_D3RF3L_40_PD611   DDR3L MSD_D3R_PDIFF_PDQSR cell  Z0=40-Ohm
MSD_D3RF3L_48_PD611   DDR3L MSD_D3R_PDIFF_PDQSR cell  Z0=48-Ohm
MSD_D3RF3L_34_PD688   DDR3L MSD_D3R_PDIFF_PDQSR cell  Z0=34-Ohm
MSD_D3RF3L_40_PD688   DDR3L MSD_D3R_PDIFF_PDQSR cell  Z0=40-Ohm
MSD_D3RF3L_48_PD688   DDR3L MSD_D3R_PDIFF_PDQSR cell  Z0=48-Ohm
MSD_D3RF3L_34_PU344   DDR3L MSD_D3R_PDIFF_PDQSR cell  Z0=34-Ohm
MSD_D3RF3L_40_PU344   DDR3L MSD_D3R_PDIFF_PDQSR cell  Z0=40-Ohm
MSD_D3RF3L_48_PU344   DDR3L MSD_D3R_PDIFF_PDQSR cell  Z0=48-Ohm
MSD_D3RF3L_34_PU393   DDR3L MSD_D3R_PDIFF_PDQSR cell  Z0=34-Ohm
MSD_D3RF3L_40_PU393   DDR3L MSD_D3R_PDIFF_PDQSR cell  Z0=40-Ohm
MSD_D3RF3L_48_PU393   DDR3L MSD_D3R_PDIFF_PDQSR cell  Z0=48-Ohm
MSD_D3RF3L_34_PU458   DDR3L MSD_D3R_PDIFF_PDQSR cell  Z0=34-Ohm
MSD_D3RF3L_40_PU458   DDR3L MSD_D3R_PDIFF_PDQSR cell  Z0=40-Ohm
MSD_D3RF3L_48_PU458   DDR3L MSD_D3R_PDIFF_PDQSR cell  Z0=48-Ohm
MSD_D3RF3L_34_PU500   DDR3L MSD_D3R_PDIFF_PDQSR cell  Z0=34-Ohm
MSD_D3RF3L_40_PU500   DDR3L MSD_D3R_PDIFF_PDQSR cell  Z0=40-Ohm
MSD_D3RF3L_48_PU500   DDR3L MSD_D3R_PDIFF_PDQSR cell  Z0=48-Ohm
MSD_D3RF3L_34_PU550   DDR3L MSD_D3R_PDIFF_PDQSR cell  Z0=34-Ohm
MSD_D3RF3L_40_PU550   DDR3L MSD_D3R_PDIFF_PDQSR cell  Z0=40-Ohm
MSD_D3RF3L_48_PU550   DDR3L MSD_D3R_PDIFF_PDQSR cell  Z0=48-Ohm
MSD_D3RF3L_34_PU611   DDR3L MSD_D3R_PDIFF_PDQSR cell  Z0=34-Ohm
MSD_D3RF3L_40_PU611   DDR3L MSD_D3R_PDIFF_PDQSR cell  Z0=40-Ohm
MSD_D3RF3L_48_PU611   DDR3L MSD_D3R_PDIFF_PDQSR cell  Z0=48-Ohm
MSD_D3RF3L_34_PU688   DDR3L MSD_D3R_PDIFF_PDQSR cell  Z0=34-Ohm
MSD_D3RF3L_40_PU688   DDR3L MSD_D3R_PDIFF_PDQSR cell  Z0=40-Ohm
MSD_D3RF3L_48_PU688   DDR3L MSD_D3R_PDIFF_PDQSR cell  Z0=48-Ohm
MSD_D3RF3L_34_PWRDWN   DDR3L MSD_D3R_PDIFF_PDQSR cell  Z0=34-Ohm
MSD_D3RF3L_40_PWRDWN   DDR3L MSD_D3R_PDIFF_PDQSR cell  Z0=40-Ohm
MSD_D3RF3L_48_PWRDWN   DDR3L MSD_D3R_PDIFF_PDQSR cell  Z0=48-Ohm
MSD_D3RFL2_34_OPEN   LPDDR2 MSD_D3R_PDIFF_PDQSR cell  Z0=34-Ohm
MSD_D3RFL2_40_OPEN   LPDDR2 MSD_D3R_PDIFF_PDQSR cell  Z0=40-Ohm
MSD_D3RFL2_48_OPEN   LPDDR2 MSD_D3R_PDIFF_PDQSR cell  Z0=48-Ohm
MSD_D3RFL2_60_OPEN   LPDDR2 MSD_D3R_PDIFF_PDQSR cell  Z0=60-Ohm
MSD_D3RFL2_80_OPEN   LPDDR2 MSD_D3R_PDIFF_PDQSR cell  Z0=80-Ohm
MSD_D3RFL_48_OPEN   LPDDR MSD_D3R_PDIFF_PDQSR cell  Z0=48-Ohm
MSD_D3RFL2_34_PD344   LPDDR2 MSD_D3R_PDIFF_PDQSR cell  Z0=34-Ohm
MSD_D3RFL2_40_PD344   LPDDR2 MSD_D3R_PDIFF_PDQSR cell  Z0=40-Ohm
MSD_D3RFL2_48_PD344   LPDDR2 MSD_D3R_PDIFF_PDQSR cell  Z0=48-Ohm
MSD_D3RFL2_60_PD344   LPDDR2 MSD_D3R_PDIFF_PDQSR cell  Z0=60-Ohm
MSD_D3RFL2_80_PD344   LPDDR2 MSD_D3R_PDIFF_PDQSR cell  Z0=80-Ohm
MSD_D3RFL_48_PD344   LPDDR MSD_D3R_PDIFF_PDQSR cell  Z0=48-Ohm
MSD_D3RFL2_34_PD393   LPDDR2 MSD_D3R_PDIFF_PDQSR cell  Z0=34-Ohm
MSD_D3RFL2_40_PD393   LPDDR2 MSD_D3R_PDIFF_PDQSR cell  Z0=40-Ohm
MSD_D3RFL2_48_PD393   LPDDR2 MSD_D3R_PDIFF_PDQSR cell  Z0=48-Ohm
MSD_D3RFL2_60_PD393   LPDDR2 MSD_D3R_PDIFF_PDQSR cell  Z0=60-Ohm
MSD_D3RFL2_80_PD393   LPDDR2 MSD_D3R_PDIFF_PDQSR cell  Z0=80-Ohm
MSD_D3RFL_48_PD393   LPDDR MSD_D3R_PDIFF_PDQSR cell  Z0=48-Ohm
MSD_D3RFL2_34_PD458   LPDDR2 MSD_D3R_PDIFF_PDQSR cell  Z0=34-Ohm
MSD_D3RFL2_40_PD458   LPDDR2 MSD_D3R_PDIFF_PDQSR cell  Z0=40-Ohm
MSD_D3RFL2_48_PD458   LPDDR2 MSD_D3R_PDIFF_PDQSR cell  Z0=48-Ohm
MSD_D3RFL2_60_PD458   LPDDR2 MSD_D3R_PDIFF_PDQSR cell  Z0=60-Ohm
MSD_D3RFL2_80_PD458   LPDDR2 MSD_D3R_PDIFF_PDQSR cell  Z0=80-Ohm
MSD_D3RFL_48_PD458   LPDDR MSD_D3R_PDIFF_PDQSR cell  Z0=48-Ohm
MSD_D3RFL2_34_PD500   LPDDR2 MSD_D3R_PDIFF_PDQSR cell  Z0=34-Ohm
MSD_D3RFL2_40_PD500   LPDDR2 MSD_D3R_PDIFF_PDQSR cell  Z0=40-Ohm
MSD_D3RFL2_48_PD500   LPDDR2 MSD_D3R_PDIFF_PDQSR cell  Z0=48-Ohm
MSD_D3RFL2_60_PD500   LPDDR2 MSD_D3R_PDIFF_PDQSR cell  Z0=60-Ohm
MSD_D3RFL2_80_PD500   LPDDR2 MSD_D3R_PDIFF_PDQSR cell  Z0=80-Ohm
MSD_D3RFL_48_PD500   LPDDR MSD_D3R_PDIFF_PDQSR cell  Z0=48-Ohm
MSD_D3RFL2_34_PD550   LPDDR2 MSD_D3R_PDIFF_PDQSR cell  Z0=34-Ohm
MSD_D3RFL2_40_PD550   LPDDR2 MSD_D3R_PDIFF_PDQSR cell  Z0=40-Ohm
MSD_D3RFL2_48_PD550   LPDDR2 MSD_D3R_PDIFF_PDQSR cell  Z0=48-Ohm
MSD_D3RFL2_60_PD550   LPDDR2 MSD_D3R_PDIFF_PDQSR cell  Z0=60-Ohm
MSD_D3RFL2_80_PD550   LPDDR2 MSD_D3R_PDIFF_PDQSR cell  Z0=80-Ohm
MSD_D3RFL_48_PD550   LPDDR MSD_D3R_PDIFF_PDQSR cell  Z0=48-Ohm
MSD_D3RFL2_34_PD611   LPDDR2 MSD_D3R_PDIFF_PDQSR cell  Z0=34-Ohm
MSD_D3RFL2_40_PD611   LPDDR2 MSD_D3R_PDIFF_PDQSR cell  Z0=40-Ohm
MSD_D3RFL2_48_PD611   LPDDR2 MSD_D3R_PDIFF_PDQSR cell  Z0=48-Ohm
MSD_D3RFL2_60_PD611   LPDDR2 MSD_D3R_PDIFF_PDQSR cell  Z0=60-Ohm
MSD_D3RFL2_80_PD611   LPDDR2 MSD_D3R_PDIFF_PDQSR cell  Z0=80-Ohm
MSD_D3RFL_48_PD611   LPDDR MSD_D3R_PDIFF_PDQSR cell  Z0=48-Ohm
MSD_D3RFL2_34_PD688   LPDDR2 MSD_D3R_PDIFF_PDQSR cell  Z0=34-Ohm
MSD_D3RFL2_40_PD688   LPDDR2 MSD_D3R_PDIFF_PDQSR cell  Z0=40-Ohm
MSD_D3RFL2_48_PD688   LPDDR2 MSD_D3R_PDIFF_PDQSR cell  Z0=48-Ohm
MSD_D3RFL2_60_PD688   LPDDR2 MSD_D3R_PDIFF_PDQSR cell  Z0=60-Ohm
MSD_D3RFL2_80_PD688   LPDDR2 MSD_D3R_PDIFF_PDQSR cell  Z0=80-Ohm
MSD_D3RFL_48_PD688   LPDDR MSD_D3R_PDIFF_PDQSR cell  Z0=48-Ohm
MSD_D3RFL2_34_PU344   LPDDR2 MSD_D3R_PDIFF_PDQSR cell  Z0=34-Ohm
MSD_D3RFL2_40_PU344   LPDDR2 MSD_D3R_PDIFF_PDQSR cell  Z0=40-Ohm
MSD_D3RFL2_48_PU344   LPDDR2 MSD_D3R_PDIFF_PDQSR cell  Z0=48-Ohm
MSD_D3RFL2_60_PU344   LPDDR2 MSD_D3R_PDIFF_PDQSR cell  Z0=60-Ohm
MSD_D3RFL2_80_PU344   LPDDR2 MSD_D3R_PDIFF_PDQSR cell  Z0=80-Ohm
MSD_D3RFL_48_PU344   LPDDR MSD_D3R_PDIFF_PDQSR cell  Z0=48-Ohm
MSD_D3RFL2_34_PU393   LPDDR2 MSD_D3R_PDIFF_PDQSR cell  Z0=34-Ohm
MSD_D3RFL2_40_PU393   LPDDR2 MSD_D3R_PDIFF_PDQSR cell  Z0=40-Ohm
MSD_D3RFL2_48_PU393   LPDDR2 MSD_D3R_PDIFF_PDQSR cell  Z0=48-Ohm
MSD_D3RFL2_60_PU393   LPDDR2 MSD_D3R_PDIFF_PDQSR cell  Z0=60-Ohm
MSD_D3RFL2_80_PU393   LPDDR2 MSD_D3R_PDIFF_PDQSR cell  Z0=80-Ohm
MSD_D3RFL_48_PU393   LPDDR MSD_D3R_PDIFF_PDQSR cell  Z0=48-Ohm
MSD_D3RFL2_34_PU458   LPDDR2 MSD_D3R_PDIFF_PDQSR cell  Z0=34-Ohm
MSD_D3RFL2_40_PU458   LPDDR2 MSD_D3R_PDIFF_PDQSR cell  Z0=40-Ohm
MSD_D3RFL2_48_PU458   LPDDR2 MSD_D3R_PDIFF_PDQSR cell  Z0=48-Ohm
MSD_D3RFL2_60_PU458   LPDDR2 MSD_D3R_PDIFF_PDQSR cell  Z0=60-Ohm
MSD_D3RFL2_80_PU458   LPDDR2 MSD_D3R_PDIFF_PDQSR cell  Z0=80-Ohm
MSD_D3RFL_48_PU458   LPDDR MSD_D3R_PDIFF_PDQSR cell  Z0=48-Ohm
MSD_D3RFL2_34_PU500   LPDDR2 MSD_D3R_PDIFF_PDQSR cell  Z0=34-Ohm
MSD_D3RFL2_40_PU500   LPDDR2 MSD_D3R_PDIFF_PDQSR cell  Z0=40-Ohm
MSD_D3RFL2_48_PU500   LPDDR2 MSD_D3R_PDIFF_PDQSR cell  Z0=48-Ohm
MSD_D3RFL2_60_PU500   LPDDR2 MSD_D3R_PDIFF_PDQSR cell  Z0=60-Ohm
MSD_D3RFL2_80_PU500   LPDDR2 MSD_D3R_PDIFF_PDQSR cell  Z0=80-Ohm
MSD_D3RFL_48_PU500   LPDDR MSD_D3R_PDIFF_PDQSR cell  Z0=48-Ohm
MSD_D3RFL2_34_PU550   LPDDR2 MSD_D3R_PDIFF_PDQSR cell  Z0=34-Ohm
MSD_D3RFL2_40_PU550   LPDDR2 MSD_D3R_PDIFF_PDQSR cell  Z0=40-Ohm
MSD_D3RFL2_48_PU550   LPDDR2 MSD_D3R_PDIFF_PDQSR cell  Z0=48-Ohm
MSD_D3RFL2_60_PU550   LPDDR2 MSD_D3R_PDIFF_PDQSR cell  Z0=60-Ohm
MSD_D3RFL2_80_PU550   LPDDR2 MSD_D3R_PDIFF_PDQSR cell  Z0=80-Ohm
MSD_D3RFL_48_PU550   LPDDR MSD_D3R_PDIFF_PDQSR cell  Z0=48-Ohm
MSD_D3RFL2_34_PU611   LPDDR2 MSD_D3R_PDIFF_PDQSR cell  Z0=34-Ohm
MSD_D3RFL2_40_PU611   LPDDR2 MSD_D3R_PDIFF_PDQSR cell  Z0=40-Ohm
MSD_D3RFL2_48_PU611   LPDDR2 MSD_D3R_PDIFF_PDQSR cell  Z0=48-Ohm
MSD_D3RFL2_60_PU611   LPDDR2 MSD_D3R_PDIFF_PDQSR cell  Z0=60-Ohm
MSD_D3RFL2_80_PU611   LPDDR2 MSD_D3R_PDIFF_PDQSR cell  Z0=80-Ohm
MSD_D3RFL_48_PU611   LPDDR MSD_D3R_PDIFF_PDQSR cell  Z0=48-Ohm
MSD_D3RFL2_34_PU688   LPDDR2 MSD_D3R_PDIFF_PDQSR cell  Z0=34-Ohm
MSD_D3RFL2_40_PU688   LPDDR2 MSD_D3R_PDIFF_PDQSR cell  Z0=40-Ohm
MSD_D3RFL2_48_PU688   LPDDR2 MSD_D3R_PDIFF_PDQSR cell  Z0=48-Ohm
MSD_D3RFL2_60_PU688   LPDDR2 MSD_D3R_PDIFF_PDQSR cell  Z0=60-Ohm
MSD_D3RFL2_80_PU688   LPDDR2 MSD_D3R_PDIFF_PDQSR cell  Z0=80-Ohm
MSD_D3RFL_48_PU688   LPDDR MSD_D3R_PDIFF_PDQSR cell  Z0=48-Ohm
MSD_D3RFL2_34_PWRDWN   LPDDR2 MSD_D3R_PDIFF_PDQSR cell  Z0=34-Ohm
MSD_D3RFL2_40_PWRDWN   LPDDR2 MSD_D3R_PDIFF_PDQSR cell  Z0=40-Ohm
MSD_D3RFL2_48_PWRDWN   LPDDR2 MSD_D3R_PDIFF_PDQSR cell  Z0=48-Ohm
MSD_D3RFL2_60_PWRDWN   LPDDR2 MSD_D3R_PDIFF_PDQSR cell  Z0=60-Ohm
MSD_D3RFL2_80_PWRDWN   LPDDR2 MSD_D3R_PDIFF_PDQSR cell  Z0=80-Ohm
MSD_D3RFL_48_PWRDWN   LPDDR MSD_D3R_PDIFF_PDQSR cell  Z0=48-Ohm
MSD_D3RF2_ODT150_OPEN   DDR2 MSD_D3R_PDIFF_PDQSR cell 150-Ohm ODT Receiver
MSD_D3RF2_ODT50_OPEN   DDR2 MSD_D3R_PDIFF_PDQSR cell 50-Ohm ODT Receiver
MSD_D3RF2_ODT75_OPEN   DDR2 MSD_D3R_PDIFF_PDQSR cell 75-Ohm ODT Receiver
MSD_D3RF2_ODTOFF_OPEN   DDR2 MSD_D3R_PDIFF_PDQSR cell ODT off Receiver
MSD_D3RF2_ODT150_PD344   DDR2 MSD_D3R_PDIFF_PDQSR cell 150-Ohm ODT Receiver
MSD_D3RF2_ODT50_PD344   DDR2 MSD_D3R_PDIFF_PDQSR cell 50-Ohm ODT Receiver
MSD_D3RF2_ODT75_PD344   DDR2 MSD_D3R_PDIFF_PDQSR cell 75-Ohm ODT Receiver
MSD_D3RF2_ODTOFF_PD344   DDR2 MSD_D3R_PDIFF_PDQSR cell ODT off Receiver
MSD_D3RF2_ODT150_PD393   DDR2 MSD_D3R_PDIFF_PDQSR cell 150-Ohm ODT Receiver
MSD_D3RF2_ODT50_PD393   DDR2 MSD_D3R_PDIFF_PDQSR cell 50-Ohm ODT Receiver
MSD_D3RF2_ODT75_PD393   DDR2 MSD_D3R_PDIFF_PDQSR cell 75-Ohm ODT Receiver
MSD_D3RF2_ODTOFF_PD393   DDR2 MSD_D3R_PDIFF_PDQSR cell ODT off Receiver
MSD_D3RF2_ODT150_PD458   DDR2 MSD_D3R_PDIFF_PDQSR cell 150-Ohm ODT Receiver
MSD_D3RF2_ODT50_PD458   DDR2 MSD_D3R_PDIFF_PDQSR cell 50-Ohm ODT Receiver
MSD_D3RF2_ODT75_PD458   DDR2 MSD_D3R_PDIFF_PDQSR cell 75-Ohm ODT Receiver
MSD_D3RF2_ODTOFF_PD458   DDR2 MSD_D3R_PDIFF_PDQSR cell ODT off Receiver
MSD_D3RF2_ODT150_PD500   DDR2 MSD_D3R_PDIFF_PDQSR cell 150-Ohm ODT Receiver
MSD_D3RF2_ODT50_PD500   DDR2 MSD_D3R_PDIFF_PDQSR cell 50-Ohm ODT Receiver
MSD_D3RF2_ODT75_PD500   DDR2 MSD_D3R_PDIFF_PDQSR cell 75-Ohm ODT Receiver
MSD_D3RF2_ODTOFF_PD500   DDR2 MSD_D3R_PDIFF_PDQSR cell ODT off Receiver
MSD_D3RF2_ODT150_PD550   DDR2 MSD_D3R_PDIFF_PDQSR cell 150-Ohm ODT Receiver
MSD_D3RF2_ODT50_PD550   DDR2 MSD_D3R_PDIFF_PDQSR cell 50-Ohm ODT Receiver
MSD_D3RF2_ODT75_PD550   DDR2 MSD_D3R_PDIFF_PDQSR cell 75-Ohm ODT Receiver
MSD_D3RF2_ODTOFF_PD550   DDR2 MSD_D3R_PDIFF_PDQSR cell ODT off Receiver
MSD_D3RF2_ODT150_PD611   DDR2 MSD_D3R_PDIFF_PDQSR cell 150-Ohm ODT Receiver
MSD_D3RF2_ODT50_PD611   DDR2 MSD_D3R_PDIFF_PDQSR cell 50-Ohm ODT Receiver
MSD_D3RF2_ODT75_PD611   DDR2 MSD_D3R_PDIFF_PDQSR cell 75-Ohm ODT Receiver
MSD_D3RF2_ODTOFF_PD611   DDR2 MSD_D3R_PDIFF_PDQSR cell ODT off Receiver
MSD_D3RF2_ODT150_PD688   DDR2 MSD_D3R_PDIFF_PDQSR cell 150-Ohm ODT Receiver
MSD_D3RF2_ODT50_PD688   DDR2 MSD_D3R_PDIFF_PDQSR cell 50-Ohm ODT Receiver
MSD_D3RF2_ODT75_PD688   DDR2 MSD_D3R_PDIFF_PDQSR cell 75-Ohm ODT Receiver
MSD_D3RF2_ODTOFF_PD688   DDR2 MSD_D3R_PDIFF_PDQSR cell ODT off Receiver
MSD_D3RF2_ODT150_PU344   DDR2 MSD_D3R_PDIFF_PDQSR cell 150-Ohm ODT Receiver
MSD_D3RF2_ODT50_PU344   DDR2 MSD_D3R_PDIFF_PDQSR cell 50-Ohm ODT Receiver
MSD_D3RF2_ODT75_PU344   DDR2 MSD_D3R_PDIFF_PDQSR cell 75-Ohm ODT Receiver
MSD_D3RF2_ODTOFF_PU344   DDR2 MSD_D3R_PDIFF_PDQSR cell ODT off Receiver
MSD_D3RF2_ODT150_PU393   DDR2 MSD_D3R_PDIFF_PDQSR cell 150-Ohm ODT Receiver
MSD_D3RF2_ODT50_PU393   DDR2 MSD_D3R_PDIFF_PDQSR cell 50-Ohm ODT Receiver
MSD_D3RF2_ODT75_PU393   DDR2 MSD_D3R_PDIFF_PDQSR cell 75-Ohm ODT Receiver
MSD_D3RF2_ODTOFF_PU393   DDR2 MSD_D3R_PDIFF_PDQSR cell ODT off Receiver
MSD_D3RF2_ODT150_PU458   DDR2 MSD_D3R_PDIFF_PDQSR cell 150-Ohm ODT Receiver
MSD_D3RF2_ODT50_PU458   DDR2 MSD_D3R_PDIFF_PDQSR cell 50-Ohm ODT Receiver
MSD_D3RF2_ODT75_PU458   DDR2 MSD_D3R_PDIFF_PDQSR cell 75-Ohm ODT Receiver
MSD_D3RF2_ODTOFF_PU458   DDR2 MSD_D3R_PDIFF_PDQSR cell ODT off Receiver
MSD_D3RF2_ODT150_PU500   DDR2 MSD_D3R_PDIFF_PDQSR cell 150-Ohm ODT Receiver
MSD_D3RF2_ODT50_PU500   DDR2 MSD_D3R_PDIFF_PDQSR cell 50-Ohm ODT Receiver
MSD_D3RF2_ODT75_PU500   DDR2 MSD_D3R_PDIFF_PDQSR cell 75-Ohm ODT Receiver
MSD_D3RF2_ODTOFF_PU500   DDR2 MSD_D3R_PDIFF_PDQSR cell ODT off Receiver
MSD_D3RF2_ODT150_PU550   DDR2 MSD_D3R_PDIFF_PDQSR cell 150-Ohm ODT Receiver
MSD_D3RF2_ODT50_PU550   DDR2 MSD_D3R_PDIFF_PDQSR cell 50-Ohm ODT Receiver
MSD_D3RF2_ODT75_PU550   DDR2 MSD_D3R_PDIFF_PDQSR cell 75-Ohm ODT Receiver
MSD_D3RF2_ODTOFF_PU550   DDR2 MSD_D3R_PDIFF_PDQSR cell ODT off Receiver
MSD_D3RF2_ODT150_PU611   DDR2 MSD_D3R_PDIFF_PDQSR cell 150-Ohm ODT Receiver
MSD_D3RF2_ODT50_PU611   DDR2 MSD_D3R_PDIFF_PDQSR cell 50-Ohm ODT Receiver
MSD_D3RF2_ODT75_PU611   DDR2 MSD_D3R_PDIFF_PDQSR cell 75-Ohm ODT Receiver
MSD_D3RF2_ODTOFF_PU611   DDR2 MSD_D3R_PDIFF_PDQSR cell ODT off Receiver
MSD_D3RF2_ODT150_PU688   DDR2 MSD_D3R_PDIFF_PDQSR cell 150-Ohm ODT Receiver
MSD_D3RF2_ODT50_PU688   DDR2 MSD_D3R_PDIFF_PDQSR cell 50-Ohm ODT Receiver
MSD_D3RF2_ODT75_PU688   DDR2 MSD_D3R_PDIFF_PDQSR cell 75-Ohm ODT Receiver
MSD_D3RF2_ODTOFF_PU688   DDR2 MSD_D3R_PDIFF_PDQSR cell ODT off Receiver
MSD_D3RF2_ODT150_PWRDWN   DDR2 MSD_D3R_PDIFF_PDQSR cell 150-Ohm ODT Receiver
MSD_D3RF2_ODT50_PWRDWN   DDR2 MSD_D3R_PDIFF_PDQSR cell 50-Ohm ODT Receiver
MSD_D3RF2_ODT75_PWRDWN   DDR2 MSD_D3R_PDIFF_PDQSR cell 75-Ohm ODT Receiver
MSD_D3RF2_ODTOFF_PWRDWN   DDR2 MSD_D3R_PDIFF_PDQSR cell ODT off Receiver
MSD_D3RF3_ODT120_OPEN   DDR3 MSD_D3R_PDIFF_PDQSR cell 120-Ohm ODT Receiver
MSD_D3RF3_ODT40_OPEN   DDR3 MSD_D3R_PDIFF_PDQSR cell 40-Ohm ODT Receiver
MSD_D3RF3_ODT60_OPEN   DDR3 MSD_D3R_PDIFF_PDQSR cell 60-Ohm ODT Receiver
MSD_D3RF3_ODTOFF_OPEN   DDR3 MSD_D3R_PDIFF_PDQSR cell ODT off Receiver
MSD_D3RF3_ODT120_PD344   DDR3 MSD_D3R_PDIFF_PDQSR cell 120-Ohm ODT Receiver
MSD_D3RF3_ODT40_PD344   DDR3 MSD_D3R_PDIFF_PDQSR cell 40-Ohm ODT Receiver
MSD_D3RF3_ODT60_PD344   DDR3 MSD_D3R_PDIFF_PDQSR cell 60-Ohm ODT Receiver
MSD_D3RF3_ODTOFF_PD344   DDR3 MSD_D3R_PDIFF_PDQSR cell ODT off Receiver
MSD_D3RF3_ODT120_PD393   DDR3 MSD_D3R_PDIFF_PDQSR cell 120-Ohm ODT Receiver
MSD_D3RF3_ODT40_PD393   DDR3 MSD_D3R_PDIFF_PDQSR cell 40-Ohm ODT Receiver
MSD_D3RF3_ODT60_PD393   DDR3 MSD_D3R_PDIFF_PDQSR cell 60-Ohm ODT Receiver
MSD_D3RF3_ODTOFF_PD393   DDR3 MSD_D3R_PDIFF_PDQSR cell ODT off Receiver
MSD_D3RF3_ODT120_PD458   DDR3 MSD_D3R_PDIFF_PDQSR cell 120-Ohm ODT Receiver
MSD_D3RF3_ODT40_PD458   DDR3 MSD_D3R_PDIFF_PDQSR cell 40-Ohm ODT Receiver
MSD_D3RF3_ODT60_PD458   DDR3 MSD_D3R_PDIFF_PDQSR cell 60-Ohm ODT Receiver
MSD_D3RF3_ODTOFF_PD458   DDR3 MSD_D3R_PDIFF_PDQSR cell ODT off Receiver
MSD_D3RF3_ODT120_PD500   DDR3 MSD_D3R_PDIFF_PDQSR cell 120-Ohm ODT Receiver
MSD_D3RF3_ODT40_PD500   DDR3 MSD_D3R_PDIFF_PDQSR cell 40-Ohm ODT Receiver
MSD_D3RF3_ODT60_PD500   DDR3 MSD_D3R_PDIFF_PDQSR cell 60-Ohm ODT Receiver
MSD_D3RF3_ODTOFF_PD500   DDR3 MSD_D3R_PDIFF_PDQSR cell ODT off Receiver
MSD_D3RF3_ODT120_PD550   DDR3 MSD_D3R_PDIFF_PDQSR cell 120-Ohm ODT Receiver
MSD_D3RF3_ODT40_PD550   DDR3 MSD_D3R_PDIFF_PDQSR cell 40-Ohm ODT Receiver
MSD_D3RF3_ODT60_PD550   DDR3 MSD_D3R_PDIFF_PDQSR cell 60-Ohm ODT Receiver
MSD_D3RF3_ODTOFF_PD550   DDR3 MSD_D3R_PDIFF_PDQSR cell ODT off Receiver
MSD_D3RF3_ODT120_PD611   DDR3 MSD_D3R_PDIFF_PDQSR cell 120-Ohm ODT Receiver
MSD_D3RF3_ODT40_PD611   DDR3 MSD_D3R_PDIFF_PDQSR cell 40-Ohm ODT Receiver
MSD_D3RF3_ODT60_PD611   DDR3 MSD_D3R_PDIFF_PDQSR cell 60-Ohm ODT Receiver
MSD_D3RF3_ODTOFF_PD611   DDR3 MSD_D3R_PDIFF_PDQSR cell ODT off Receiver
MSD_D3RF3_ODT120_PD688   DDR3 MSD_D3R_PDIFF_PDQSR cell 120-Ohm ODT Receiver
MSD_D3RF3_ODT40_PD688   DDR3 MSD_D3R_PDIFF_PDQSR cell 40-Ohm ODT Receiver
MSD_D3RF3_ODT60_PD688   DDR3 MSD_D3R_PDIFF_PDQSR cell 60-Ohm ODT Receiver
MSD_D3RF3_ODTOFF_PD688   DDR3 MSD_D3R_PDIFF_PDQSR cell ODT off Receiver
MSD_D3RF3_ODT120_PU344   DDR3 MSD_D3R_PDIFF_PDQSR cell 120-Ohm ODT Receiver
MSD_D3RF3_ODT40_PU344   DDR3 MSD_D3R_PDIFF_PDQSR cell 40-Ohm ODT Receiver
MSD_D3RF3_ODT60_PU344   DDR3 MSD_D3R_PDIFF_PDQSR cell 60-Ohm ODT Receiver
MSD_D3RF3_ODTOFF_PU344   DDR3 MSD_D3R_PDIFF_PDQSR cell ODT off Receiver
MSD_D3RF3_ODT120_PU393   DDR3 MSD_D3R_PDIFF_PDQSR cell 120-Ohm ODT Receiver
MSD_D3RF3_ODT40_PU393   DDR3 MSD_D3R_PDIFF_PDQSR cell 40-Ohm ODT Receiver
MSD_D3RF3_ODT60_PU393   DDR3 MSD_D3R_PDIFF_PDQSR cell 60-Ohm ODT Receiver
MSD_D3RF3_ODTOFF_PU393   DDR3 MSD_D3R_PDIFF_PDQSR cell ODT off Receiver
MSD_D3RF3_ODT120_PU458   DDR3 MSD_D3R_PDIFF_PDQSR cell 120-Ohm ODT Receiver
MSD_D3RF3_ODT40_PU458   DDR3 MSD_D3R_PDIFF_PDQSR cell 40-Ohm ODT Receiver
MSD_D3RF3_ODT60_PU458   DDR3 MSD_D3R_PDIFF_PDQSR cell 60-Ohm ODT Receiver
MSD_D3RF3_ODTOFF_PU458   DDR3 MSD_D3R_PDIFF_PDQSR cell ODT off Receiver
MSD_D3RF3_ODT120_PU500   DDR3 MSD_D3R_PDIFF_PDQSR cell 120-Ohm ODT Receiver
MSD_D3RF3_ODT40_PU500   DDR3 MSD_D3R_PDIFF_PDQSR cell 40-Ohm ODT Receiver
MSD_D3RF3_ODT60_PU500   DDR3 MSD_D3R_PDIFF_PDQSR cell 60-Ohm ODT Receiver
MSD_D3RF3_ODTOFF_PU500   DDR3 MSD_D3R_PDIFF_PDQSR cell ODT off Receiver
MSD_D3RF3_ODT120_PU550   DDR3 MSD_D3R_PDIFF_PDQSR cell 120-Ohm ODT Receiver
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| Models and submodels in the file (581): io8_ft_et_fs_1v2 (I/O), io8_ft_et_hs_1v2 (I/O), io8_ft_et_hslv_fs_1v2 (I/O), io8_ft_et_hslv_hs_1v2 (I/O), io8_ft_et_hslv_ls_1v2 (I/O), io8_ft_et_hslv_ms_1v2 (I/O), io8_ft_et_ls_1v2 (I/O), io8_ft_et_ms_1v2 (I/O), io8_ft_fs_1v2 (I/O), io8_ft_hs_1v2 (I/O), io8_ft_hslv_fs_1v2 (I/O), io8_ft_hslv_hs_1v2 (I/O), io8_ft_hslv_ls_1v2 (I/O), io8_ft_hslv_ms_1v2 (I/O), io8_ft_i2c_1v2 (I/O_open_drain), io8_ft_i2c_hslv_1v2 (I/O_open_drain), io8_ft_ls_1v2 (I/O), io8_ft_ms_1v2 (I/O), isudqf_1v2 (Input), io8_ft_et_fs_1v8 (I/O), io8_ft_et_hs_1v8 (I/O), io8_ft_et_hslv_fs_1v8 (I/O), io8_ft_et_hslv_hs_1v8 (I/O), io8_ft_et_hslv_ls_1v8 (I/O), io8_ft_et_hslv_ms_1v8 (I/O), io8_ft_et_ls_1v8 (I/O), io8_ft_et_ms_1v8 (I/O), io8_ft_fs_1v8 (I/O), io8_ft_hs_1v8 (I/O), io8_ft_hslv_fs_1v8 (I/O), io8_ft_hslv_hs_1v8 (I/O), io8_ft_hslv_ls_1v8 (I/O), io8_ft_hslv_ms_1v8 (I/O), io8_ft_i2c_1v8 (I/O_open_drain), io8_ft_i2c_hslv_1v8 (I/O_open_drain), io8_ft_ls_1v8 (I/O), io8_ft_ms_1v8 (I/O), isudqf_1v8 (Input), io8_ft_et_hslv_fs_2v5 (I/O), io8_ft_et_hslv_hs_2v5 (I/O), io8_ft_et_hslv_ls_2v5 (I/O), io8_ft_et_hslv_ms_2v5 (I/O), io8_ft_hslv_fs_2v5 (I/O), io8_ft_hslv_hs_2v5 (I/O), io8_ft_hslv_ls_2v5 (I/O), io8_ft_hslv_ms_2v5 (I/O), io8_ft_i2c_hslv_2v5 (I/O_open_drain), io8_ft_et_fs_3v3 (I/O), io8_ft_et_hs_3v3 (I/O), io8_ft_et_ls_3v3 (I/O), io8_ft_et_ms_3v3 (I/O), io8_ft_fs_3v3 (I/O), io8_ft_hs_3v3 (I/O), io8_ft_i2c_3v3 (I/O_open_drain), io8_ft_ls_3v3 (I/O), io8_ft_ms_3v3 (I/O), io8usb_ft_hs_3v3 (I/O), io8usb_ft_ls_3v3 (I/O), isudqf_3v3 (Input), MSD_D3RF2_18 (I/O), MSD_D3RF2_40 (I/O), MSD_D3RF2_48 (I/O), MSD_D3RF2_ODT150 (Input), MSD_D3RF2_ODT50 (Input), MSD_D3RF2_ODT75 (Input), MSD_D3RF2_ODTOFF (Input), MSD_D3RF3_34 (I/O), MSD_D3RF3_40 (I/O), MSD_D3RF3_48 (I/O), MSD_D3RF3L_34 (I/O), MSD_D3RF3L_40 (I/O), MSD_D3RF3L_48 (I/O), MSD_D3RF3L_ODT120 (Input), MSD_D3RF3L_ODT40 (Input), MSD_D3RF3L_ODT60 (Input), MSD_D3RF3L_ODTOFF (Input), MSD_D3RF3_ODT120 (Input), MSD_D3RF3_ODT40 (Input), MSD_D3RF3_ODT60 (Input), MSD_D3RF3_ODTOFF (Input)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
